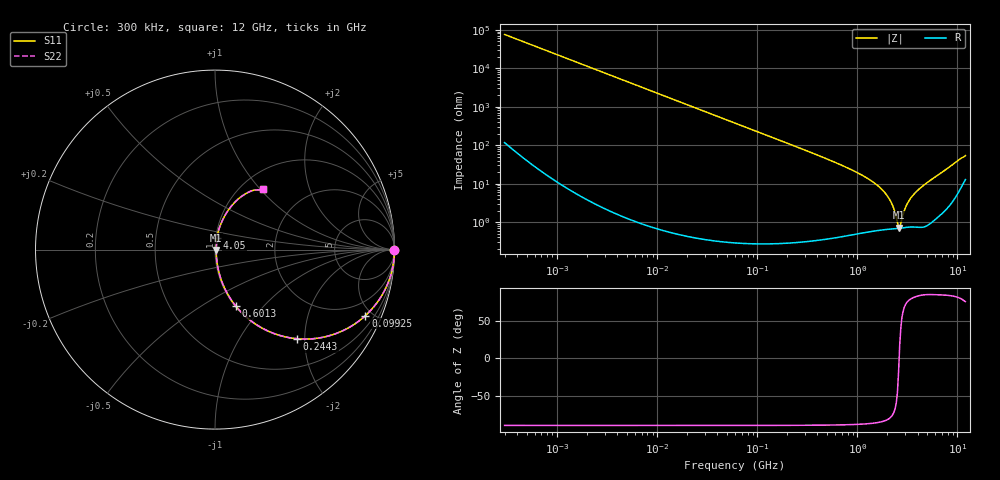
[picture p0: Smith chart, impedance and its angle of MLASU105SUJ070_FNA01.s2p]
! MLASU105SUJ070_FNA01  S-PARAMETER MODEL  ( General Type )
! Model Generated by TAIYO YUDEN Corporation (http://www.ty-top.com)
! Version 2.0
! TAIYO YUDEN Control No. 120810
! Copyright(c) 2011 TAIYO YUDEN CO.,LTD. All Rights Reserved.
! Product Description (link to TY-COMPAS)
! https://ds.yuden.co.jp/TYCOMPAS/or/detail?pn=MLASU105SUJ070DFNA01&u=M
! Products Name : Multilayer Ceramic Capacitors
! Characteristics :
!  Capacitance : 7 pF , Rated Voltage : 50V , TCC : UJ / U2J
!  Case Size : 1.0 x 0.5 / 0.039 x 0.02 [mm/inch] , Thickness : 0.5 / 0.02 [mm/inch]
!  (Conditions: Temperature = 25 degC , DC Bias Current/Voltage = 0A / 0V)
! External Node Assignments :
!  1  o---| |---o  2
! GND o---------o GND
! Frequency Range : 0.3MHz  -  12000MHz  [ 401 STEP ]
# MHz S RI R 50
! Freq[MHz].  S11 Real  S11 Imag  S21 Real  S21 Imag  S12 Real  S12 Imag  S22 Real  S22 Imag
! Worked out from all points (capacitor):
!   401 points, 300 kHz to 12 GHz, reference 50 ohm
!   read as one part in series: C = 7.03 pF near 316.3 kHz
!   lowest |Z| = 722 mohm at 2.582 GHz (marker M1)
!   series resonance near 2.616 GHz, so ESL is about 530 pH
!   S11 on the Smith chart (normalised r, x): 300 kHz: open; 99.25 MHz: 1.01, -4.55; 244.3 MHz: 1.01, -1.84; 601.3 MHz: 1.01, -0.71; 4.05 GHz: 1.01, +0.14; 12 GHz: 1.25, +1.04
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0.3  1 -0.00133  3.8e-06 0.00133  3.8e-06 0.00133  1 -0.00133
1.769972  0.9999 -0.00782  6.39e-05 0.00782  6.39e-05 0.00782  0.9999 -0.00782
10.44266  0.9979 -0.046  0.00214 0.046  0.00214 0.046  0.9979 -0.046
27.10171  0.9858 -0.118  0.0142 0.118  0.0142 0.118  0.9858 -0.118
60  0.9341 -0.2477  0.0659 0.2477  0.0659 0.2477  0.9341 -0.2477
99.25425  0.838 -0.3678  0.162 0.3678  0.162 0.3678  0.838 -0.3678
164.1901  0.6531 -0.475  0.3469 0.475  0.3469 0.475  0.6531 -0.475
244.3004  0.4577 -0.4966  0.5423 0.4966  0.5423 0.4966  0.4577 -0.4966
353.9943  0.2837 -0.4482  0.7163 0.4482  0.7163 0.4482  0.2837 -0.4482
601.3112  0.1155 -0.3142  0.8845 0.3142  0.8845 0.3142  0.1155 -0.3142
1366.97  0.0197 -0.1174  0.9803 0.1174  0.9803 0.1174  0.0197 -0.1174
1735.023  0.0114 -0.0719  0.9886 0.0719  0.9886 0.0719  0.0114 -0.0719
2088.533  0.00805 -0.0389  0.9919 0.0389  0.9919 0.0389  0.00805 -0.0389
2261.293  0.00729 -0.0251  0.9927 0.0251  0.9927 0.0251  0.00729 -0.0251
2514.07  0.00684 -0.00696  0.9932 0.00696  0.9932 0.00696  0.00684 -0.00696
2581.562  0.00682 -0.0022  0.9932 0.0022  0.9932 0.0022  0.00682 -0.0022
2722.03  0.00699 0.00619  0.993 -0.00619  0.993 -0.00619  0.00699 0.00619
3026.31  0.00772 0.0224  0.9923 -0.0224  0.9923 -0.0224  0.00772 0.0224
3276.641  0.00858 0.0346  0.9914 -0.0346  0.9914 -0.0346  0.00858 0.0346
4050.141  0.0118 0.0671  0.9882 -0.0671  0.9882 -0.0671  0.0118 0.0671
7648.807  0.0685 0.2117  0.9315 -0.2117  0.9315 -0.2117  0.0685 0.2117
12000  0.2683 0.337  0.7317 -0.337  0.7317 -0.337  0.2683 0.337
